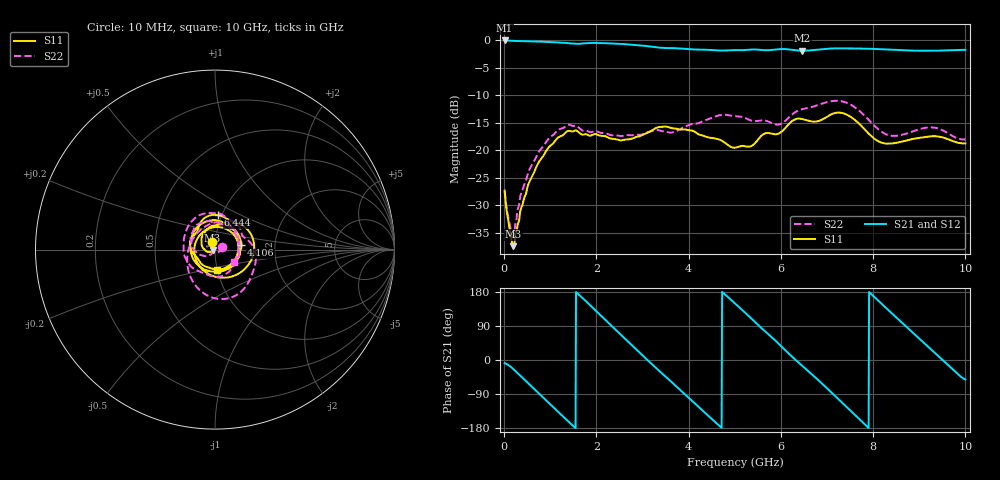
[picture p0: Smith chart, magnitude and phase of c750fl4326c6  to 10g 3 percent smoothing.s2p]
!Agilent Technologies,N5234A,MY52241123,A.10.00.00
!Agilent N5234A: A.10.00.00
!Date: Monday, May 06, 2019 14:04:20
!Correction: S11(Full 2 Port(1,2))
!S21(Full 2 Port(1,2))
!S12(Full 2 Port(1,2))
!S22(Full 2 Port(1,2))
!S2P File: Measurements: S11, S21, S12, S22:
# Hz S  dB  R 50
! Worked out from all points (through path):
!   1001 points, 10 MHz to 10 GHz, reference 50 ohm
!   highest |S21| = -0.06 dB at 10 MHz (marker M1); lowest = -1.9 dB at 6.464 GHz (marker M2)
!   group delay of S21, straight-line fit = 314 ps
!   lowest |S11| = -37.4 dB at 199.8 MHz (marker M3), VSWR 1.03, Z = 48.7 - j0.218 ohm
!   |S11| at or under -10 dB: start of sweep to end of sweep
!   |S22| runs from -35.5 to -11.0 dB; largest |S21 - S12| = 0.0015
!   S11 on the Smith chart (normalised r, x): 10 MHz: 0.96, +0.08; 4.106 GHz: 1.34, +0.07; 6.444 GHz: 0.96, +0.38; 10 GHz: 0.99, -0.23
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1e7  -27.28 112.9  -0.06 -8.0  -0.07 -8.0  -27.45 21.3
1.9981e8  -37.38 -170.5  -0.14 -24.0  -0.14 -24.0  -35.49 -110.6
8.6914e8  -20.72 145.0  -0.30 -101.7  -0.30 -101.7  -19.02 -176.9
1.29871e9  -17.06 81.8  -0.48 -151.4  -0.47 -151.5  -15.86 138.9
1.67833e9  -17.12 24.6  -0.63 166.2  -0.63 166.2  -16.33 94.7
2.4076e9  -17.96 -76.3  -0.64 80.9  -0.64 80.9  -17.28 13.9
2.89711e9  -17.51 -162.4  -0.94 24.0  -0.94 24.0  -17.16 -39.0
3.34666e9  -15.79 118.4  -1.36 -27.1  -1.36 -27.1  -16.34 -84.8
4.1059e9  -16.50 9.6  -1.70 -111.6  -1.70 -111.6  -15.12 -174.4
4.55545e9  -17.82 -44.9  -1.83 -161.6  -1.83 -161.6  -13.91 133.7
5.005e9  -19.52 -108.4  -1.81 149.1  -1.81 149.1  -13.81 93.5
5.66434e9  -16.90 163.8  -1.83 74.9  -1.83 74.9  -14.61 46.5
6.09391e9  -15.96 124.5  -1.63 25.9  -1.63 25.9  -14.66 18.4
6.44356e9  -14.29 85.0  -1.93 -13.1  -1.93 -13.1  -12.57 -15.1
6.46354e9  -14.32 82.9  -1.94 -15.2  -1.93 -15.2  -12.53 -17.0
6.67333e9  -14.77 65.7  -1.84 -37.8  -1.83 -37.8  -12.13 -33.6
7.33267e9  -13.23 -0.1  -1.50 -113.6  -1.50 -113.6  -11.12 -82.7
7.84216e9  -16.41 -89.6  -1.55 -172.4  -1.55 -172.5  -13.94 -134.0
8.34166e9  -18.78 162.6  -1.72 130.3  -1.73 130.3  -17.25 155.6
8.79121e9  -18.08 92.5  -1.89 79.8  -1.89 79.7  -16.76 100.9
9.29071e9  -17.44 33.5  -1.93 24.2  -1.93 24.1  -15.85 58.9
1e10  -18.73 -84.7  -1.77 -51.6  -1.77 -51.6  -18.04 -33.3
